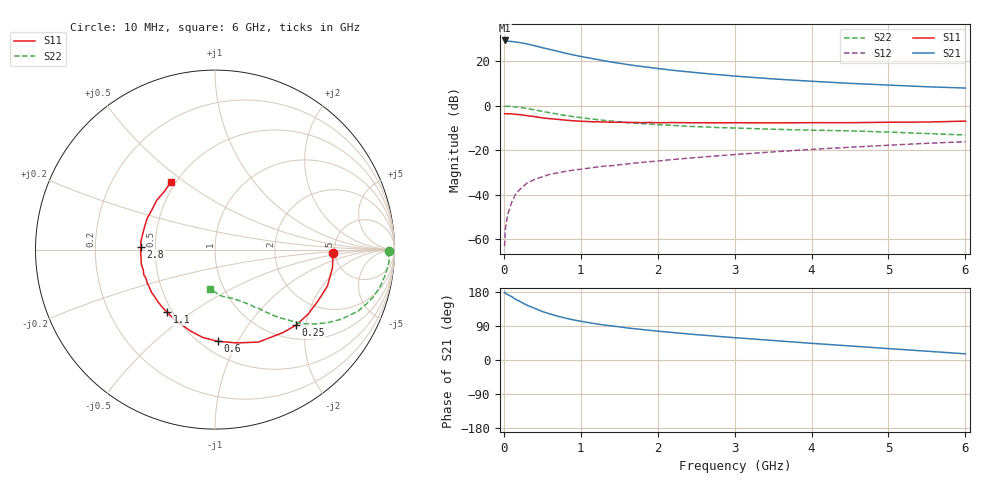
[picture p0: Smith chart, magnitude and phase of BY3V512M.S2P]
! SIEMENS Small Signal Semiconductors
! BFY420
! Si NPN RF SIEGET Grounded Emitter Transistor in MICRO-X
! VCE = 3.5 V  IC = 12 mA
! Common Emitter S-Parameters:  October  1996
# GHz  S  MA  R  50
!  f  S11  S21  S12  S22
! GHz  MAG  ANG  MAG  ANG  MAG  ANG  MAG  ANG
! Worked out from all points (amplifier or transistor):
!   36 points, 10 MHz to 6 GHz, reference 50 ohm
!   highest |S21| = 29.3 dB at 10 MHz (marker M1)
!   |S21| within 3 dB of that: start of sweep to 471.9 MHz
!   unconditionally stable (mu >= 1): start of sweep to 11.78 MHz; 2.385 GHz to end of sweep
!   at 250 MHz: K = 0.23, MSG = 32.2 dB, |S12| = -36.3 dB
!   at 1.4 GHz: K = 0.80, MSG = 23.3 dB, |S12| = -27.0 dB
!   at 6 GHz: K = 1.08, MAG = 10.4 dB, |S12| = -16.2 dB
!   S11 on the Smith chart (normalised r, x): 10 MHz: 4.86, -0.34; 250 MHz: 1.29, -1.76; 600 MHz: 0.60, -0.83; 1.1 GHz: 0.47, -0.40; 2.8 GHz: 0.42, +0.02; 6 GHz: 0.47, +0.45
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0.01  0.6604 -1.7  29.25 178.7  0.0007 49.9  0.9705 -0.6
0.02  0.6579 -4.0  29.13 176.2  0.0017 72.3  0.9663 -1.4
0.05  0.6623 -8.8  28.14 172.7  0.0036 74.5  0.9721 -4.0
0.1  0.6586 -18.0  27.79 167.4  0.0066 77.0  0.9598 -8.4
0.15  0.6414 -26.3  27.01 160.5  0.0101 74.3  0.9434 -12.5
0.2  0.6315 -34.6  26.33 155.7  0.0128 73.4  0.9231 -16.3
0.25  0.6176 -43.0  25.46 149.8  0.0153 70.0  0.8951 -19.9
0.3  0.5983 -50.4  24.43 144.7  0.0182 67.2  0.8682 -23.2
0.4  0.5695 -64.8  22.3 136.4  0.022 62.6  0.8057 -28.7
0.5  0.5336 -77.0  20.12 127.9  0.0253 60.2  0.7469 -33.1
0.6  0.5115 -88.1  18.37 121.6  0.0288 57.5  0.6931 -36.7
0.8  0.4748 -106.3  15.16 110.5  0.0335 53.4  0.6045 -42.0
0.9  0.4591 -113.3  13.86 106.1  0.0357 53.3  0.5698 -43.7
1.1  0.4403 -127.4  11.9 98.7  0.0395 52.8  0.5139 -47.1
1.3  0.4314 -137.0  10.25 92.6  0.0438 52.1  0.4699 -49.4
1.6  0.4214 -150.5  8.456 84.7  0.0492 52.0  0.4194 -52.7
2.2  0.4186 -168.7  6.246 72.4  0.062 51.7  0.3616 -58.1
2.8  0.4133 177.8  4.965 62.1  0.0753 49.9  0.3221 -63.0
3.5  0.4119 164.3  4.004 51.5  0.0919 46.9  0.2966 -68.4
4.5  0.4158 147.4  3.182 37.1  0.1166 40.6  0.273 -77.2
5.5  0.4301 130.6  2.668 23.2  0.1429 32.7  0.2372 -89.7
6  0.4508 122.9  2.494 16.3  0.1556 28.3  0.2201 -97.8
